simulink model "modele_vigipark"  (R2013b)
settings: Solver=ode23  StartTime=0.0  StopTime=0  MaxStep=0.1  RelTol=1e-4
undefined symbols (not defined in the file): Acid, Lead
libraries: fl_lib x6, nesl_utility x4, powerlib x2, electricdrivelib x1

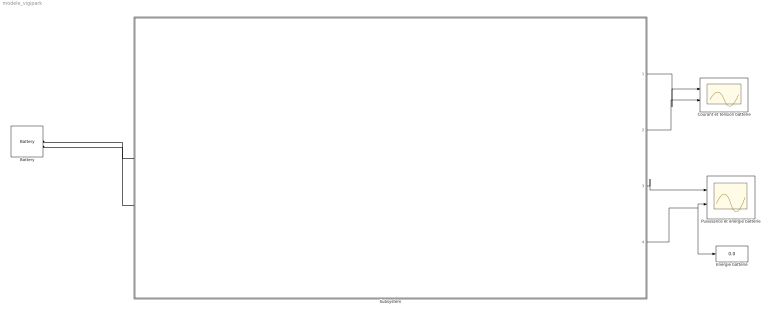
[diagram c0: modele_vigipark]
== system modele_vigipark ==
  Battery : electricdrivelib/Extra Sources/Battery  BatType=Lead-Acid  ShowDetailedParameters=off  NomV=0  NomQ=0  SOC=100  PresetModel=on  MaxQ=7.2917  FullV=13.5013  Dis_rate=1.4  R=0.017714  Normal_OP=2.1719  expZone="[12.6243    0.0233333]"  Dis_Char=off  current=[1.5 3]  Units=Time  Batt_Tr=30
  Courant et tension batterie : Scope  NumInputPorts=2
  Energie batterie : Display
  Puisssance et énergie batterie : Scope  NumInputPorts=2
  Subsystem : Subsystem
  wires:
  Subsystem/4(Out5) -> Puisssance et énergie batterie/2, Energie batterie/1
  Subsystem/1(Out2) -> Courant et tension batterie/1
  Subsystem/2(Out3) -> Courant et tension batterie/2
  Subsystem/3(Out4) -> Puisssance et énergie batterie/1
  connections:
  Battery/LConn1 -- Subsystem/LConn1
  Battery/LConn2 -- Subsystem/LConn2

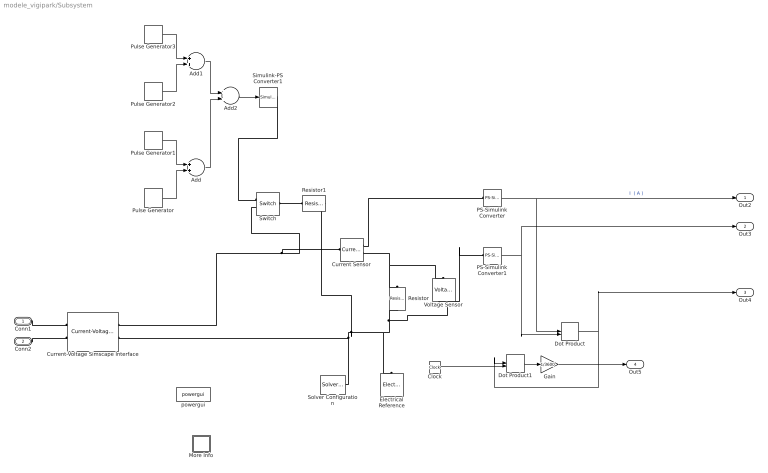
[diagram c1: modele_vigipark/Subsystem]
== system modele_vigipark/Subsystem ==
  Add : Sum
  Add1 : Sum
  Add2 : Sum
  Clock : Clock
  Current Sensor : fl_lib/Electrical/Electrical Sensors/Current Sensor  i1_Log=off  v1_Log=off  LocalVarNames=|i1|v1  LocalVarDescs=|i1|v1  LocalVarLogging=[0 0]
  Current-Voltage Simscape Interface : powerlib/Interface Elements/Current-Voltage Simscape Interface  DFT=on  FMode=Low pass filter (continuous)  T=1e-6  Ts=50e-6  i0=0  v0=0  Sd=Simscape side  Measurements=off
  Dot Product : DotProduct
  Dot Product1 : DotProduct
  Electrical Reference : fl_lib/Electrical/Electrical Elements/Electrical Reference  i_Log=off  LocalVarNames=|i  LocalVarDescs=|i  LocalVarLogging=0
  Gain : Gain  Gain=1/3600
  More Info : Subsystem
  PS-Simulink Converter : nesl_utility/PS-Simulink Converter  PhysicalDomain=network_engine_domain  SubClassName=ps_output  LeftPortType=input  RightPortType=output  PseudoPeriodic=off  Frequencies=[]  Unit=1  AffineConversion=off
  PS-Simulink Converter1 : nesl_utility/PS-Simulink Converter  PhysicalDomain=network_engine_domain  SubClassName=ps_output  LeftPortType=input  RightPortType=output  PseudoPeriodic=off  Frequencies=[]  Unit=1  AffineConversion=off
  Pulse Generator : DiscretePulseGenerator  PulseType=Time based  Amplitude=5  Period=86400  PulseWidth=0.0087  PhaseDelay=72015
  Pulse Generator1 : DiscretePulseGenerator  PulseType=Time based  Amplitude=5  Period=86400  PulseWidth=0.0087  PhaseDelay=72000
  Pulse Generator2 : DiscretePulseGenerator  PulseType=Time based  Amplitude=5  Period=86400  PulseWidth=0.0087  PhaseDelay=36015
  Pulse Generator3 : DiscretePulseGenerator  PulseType=Time based  Amplitude=5  Period=86400  PulseWidth=0.0087  PhaseDelay=36000
  Resistor : fl_lib/Electrical/Electrical Elements/Resistor  R=59 Ohm  i_Log=off  v_Log=off  LocalVarNames=|i|v  LocalVarDescs=|i|v  LocalVarLogging=[0 0]
  Resistor1 : fl_lib/Electrical/Electrical Elements/Resistor  R=103 Ohm  i_Log=off  v_Log=off  LocalVarNames=|i|v  LocalVarDescs=|i|v  LocalVarLogging=[0 0]
  Simulink-PS Converter1 : nesl_utility/Simulink-PS Converter  PhysicalDomain=network_engine_domain  SubClassName=ps_input  LeftPortType=input  RightPortType=output  PseudoPeriodic=off  Frequencies=[]  NoiseDistribution=none  NoiseParameters=[]  Unit=1  AffineConversion=off  InputFiltering=off  SimscapeFilterOrder=1  InputFilterTimeConstant=0.001  UdotUserProvided=1
  Solver Configuration : nesl_utility/Solver Configuration  PhysicalDomain=network_engine_domain  SubClassName=solver  LeftPortType=input  RightPortType=generic  Accelerate=off  Tones=[]  Harmonics=[]  SimulateNoise=off  Profile=off  UseLocalSampling=off  EnableSwitchedLinearOptims=on  FrequencyDomain=off  UseCCode=off  RelTol=0.001  AbsTol=1e-06  MinStep=1e-09  ToWorkspace=off  DoDC=off  ResidualTolerance=1e-9  UseLocalSolver=off  LocalSolverChoice=NE_BACKWARD_EULER_ADVANCER  LocalSolverSampleTime=.001  DoFixedCost=off  MaxNonlinIter=3  MaxModeIter=2  LinearAlgebra=Sparse  DelaysMemoryBudget=1024
  Switch : fl_lib/Electrical/Electrical Elements/Switch  R_closed=0.01 Ohm  G_open=1e-8 1/Ohm  Threshold=0  i_Log=off  v_Log=off  LocalVarNames=|i|v  LocalVarDescs=|i|v  LocalVarLogging=[0 0]
  Voltage Sensor : fl_lib/Electrical/Electrical Sensors/Voltage Sensor  i1_Log=off  v1_Log=off  LocalVarNames=|i1|v1  LocalVarDescs=|i1|v1  LocalVarLogging=[0 0]
  powergui : powerlib/powergui  SimulationMode=Continuous  SolverType=Tustin  SampleTime=0.001  frequency=60  SPID=off  DisableSnubberDevices=off  DisableRonSwitches=off  DisableVfSwitches=off  SwTol=0  Interpol=off  DisplayEquations=off  frequencyindice=0  Pbase=100e6  ErrMax=1e-4  Iterations=50  UnitsV=kV  UnitsW=MW  FunctionMessages=off  echomessages=off  HookPort=off  EnableUseOfTLC=off  x0status=blocks  RestoreLinks=warning  ResistiveCurrentMeasurement=off  Frange=[0:2:500]  Ylog=off  Xlog=on  ShowGrid=off  save=off  variable=ZData  ZoomFFT=on  StartTime=0.0  cycles=1  DisplayStyle=1  fundamental=60  FreqAxis=off  MaxFrequency=1000  frequencyindicesteady=1  RmsSteady=1  display=off  Ts=0  methode=off
  Conn1 : PMIOPort  Port=1  Side=Left
  Conn2 : PMIOPort  Port=2  Side=Left
  Out2 : Outport
  Out3 : Outport  Port=2
  Out4 : Outport  Port=3
  Out5 : Outport  Port=4
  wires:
  Add1/1 -> Add2/1
  Pulse Generator/1 -> Add/2
  Add/1 -> Add2/2
  Add2/1 -> Simulink-PS Converter1/1
  Clock/1 -> Dot Product1/2
  Pulse Generator1/1 -> Add/1
  Dot Product1/1 -> Gain/1
  PS-Simulink Converter/1 -> Out2/1, Dot Product/1  "I  ( A )"
  PS-Simulink Converter1/1 -> Out3/1, Dot Product/2
  Gain/1 -> Out5/1
  Pulse Generator3/1 -> Add1/1
  Pulse Generator2/1 -> Add1/2
  Dot Product/1 -> Out4/1, Dot Product1/1
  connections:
  Conn1/RConn1 -- Current-Voltage Simscape Interface/LConn1
  Resistor1/LConn1 -- Switch/LConn1
  Voltage Sensor/RConn1 -- PS-Simulink Converter1/LConn1
  Conn2/RConn1 -- Current-Voltage Simscape Interface/LConn2
  Current-Voltage Simscape Interface/RConn1 -- Switch/RConn2 -- Current Sensor/LConn1
  Simulink-PS Converter1/RConn1 -- Switch/RConn1
  Current Sensor/RConn2 -- Resistor/LConn1 -- Voltage Sensor/LConn1
  Current Sensor/RConn1 -- PS-Simulink Converter/LConn1
  Current-Voltage Simscape Interface/RConn2 -- Resistor1/RConn1 -- Resistor/RConn1 -- Voltage Sensor/RConn2 -- Electrical Reference/LConn1 -- Solver Configuration/RConn1

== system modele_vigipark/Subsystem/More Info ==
